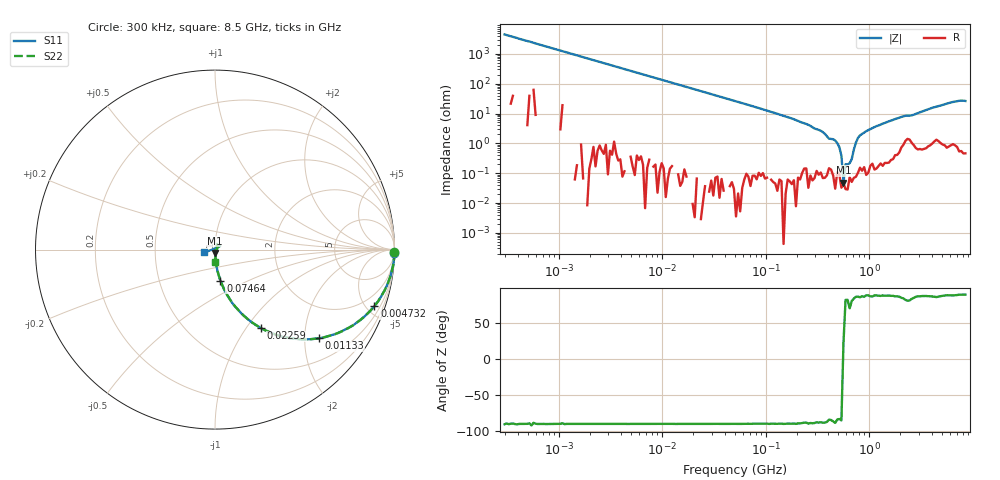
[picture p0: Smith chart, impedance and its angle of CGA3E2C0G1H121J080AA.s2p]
! S-parameter Generated by TDK Corporation
! Copyright(C) 2015 TDK Corporation.
! All Rights Reserved.
! TDK P/N: CGA3E2C0G1H121J080AA (Multilayer Ceramic Chip Capacitors)
! Property: C=120pF
! Size(LxWxT): 1.6x0.8x0.8mm, 0.063x0.031x0.031inches
! Model Type: s2p (Touchstone File Format Version 1.0)
! Frequency: DC=Yes Start=0.3MHz Stop=8500MHz 225points Log-sweep
! Note:
! Model Generated on Jun. 23, 2015
! Hash(MD5):
! Port Assignments:
!  1 ---| |--- 2
! Applicable Conditions:
!  Temperature = 25 degC
!  DC Bias Voltage = 0 V
!  Small Signal Operation
! Terms and conditions regarding TDK Simulation Models
! (1)This simulation model is being provided solely for informational purposes. Please refer to the specifications of the products in terms of detailed characteristics of such products.
! (2)In no event shall TDK Corporation of any of its subsidiaries be liable for any loss or damage arising, directly or indirectly,
!  From any information contained in this simulation model, including, but not limited to loss or damages arising from any inaccuracies, omissions or errors in connection with such information.
! (3)Any and all copyrights on this simulation model are owned by TDK Corporation.
!  Duplication or redistribution of this simulation model without prior written permission from TDK Corporation is prohibited.
! (4)This simulation model is subject to any modification or change without any prior notice.
! (5)Neither TDK Corporation nor any of its subsidiaries shall make any warranty, express or implied,
!  Including but not limited to the correctness, implied warranties of merchantability and fitness for a particular purpose with respect to this simulation models.
! (6)The use of this simulation model shall be deemed to have consented to the terms and conditions hereof.
# MHz S MA R 50
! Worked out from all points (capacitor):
!   224 points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, 300 kHz to 8.5 GHz, reference 50 ohm
!   read as one part in series: C = 120 pF near 314.1 kHz
!   lowest |Z| = 48.5 mohm at 564.2 MHz (marker M1)
!   series resonance near 563.1 MHz, so ESL is about 670 pH
!   S11 on the Smith chart (normalised r, x): 300 kHz: 1, -99; 4.732 MHz: 1.00, -5.62; 11.33 MHz: 1.00, -2.35; 22.59 MHz: 1.00, -1.18; 74.64 MHz: 1.00, -0.36; 8.5 GHz: 0.88, -0.03
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0.3  0.9997 -1.2  0.02245 89.5  0.02245 88.6  0.9997 -0.7
1.72111  0.9914 -7.3  0.1282 82.7  0.1281 82.6  0.9917 -7.3
4.732045  0.9424 -19.6  0.3346 70.5  0.3346 70.4  0.9424 -19.5
9.430415  0.8163 -35.3  0.5776 54.6  0.5776 54.7  0.8163 -35.3
11.33425  0.762 -40.5  0.6473 49.5  0.6473 49.6  0.7622 -40.4
22.58783  0.5074 -59.7  0.8607 30.4  0.8609 30.4  0.5083 -59.6
51.67171  0.2493 -75.7  0.9682 14.3  0.9683 14.2  0.2493 -75.7
74.64084  0.175 -80.1  0.9837 9.8  0.9837 9.9  0.1747 -79.9
283.1228  0.04381 -87.7  0.9987 1.5  0.9981 1.5  0.04347 -88.0
564.2308  0.0194 -89.4  0.9997 -1.1  0.9979 -1.1  0.01841 -93.9
1232.735  0.004887 -102.5  0.996 -4.8  0.9991 -4.8  0.005548 -65.9
1551.304  0.002409 -111.9  0.9973 -6.4  0.9964 -6.4  0.004851 -50.1
1864.484  0.001025 -37.0  0.9944 -8.0  0.9948 -7.8  0.005189 -25.3
2044.041  0.003643 1.9  0.9906 -8.8  0.991 -8.8  0.007259 -8.9
2346.313  0.01165 -28.5  0.9842 -9.9  0.9849 -9.8  0.01477 -23.1
2693.286  0.01059 -67.9  0.9905 -11.0  0.9892 -10.9  0.01247 -52.8
3237.012  0.004325 -30.5  0.9935 -13.4  0.9925 -13.4  0.006866 -10.1
4265.177  0.02119 37.5  0.9884 -17.9  0.9878 -17.9  0.02111 39.0
6161.135  0.03657 38.9  0.9875 -25.9  0.9868 -25.8  0.0341 68.7
7404.957  0.02229 44.2  0.9902 -30.7  0.9897 -30.7  0.0206 62.3
7753.325  0.008159 73.1  0.9892 -32.2  0.9904 -32.2  0.00889 12.0
8500  0.06295 -165.7  0.9848 -35.2  0.9881 -35.1  0.06986 -88.8
